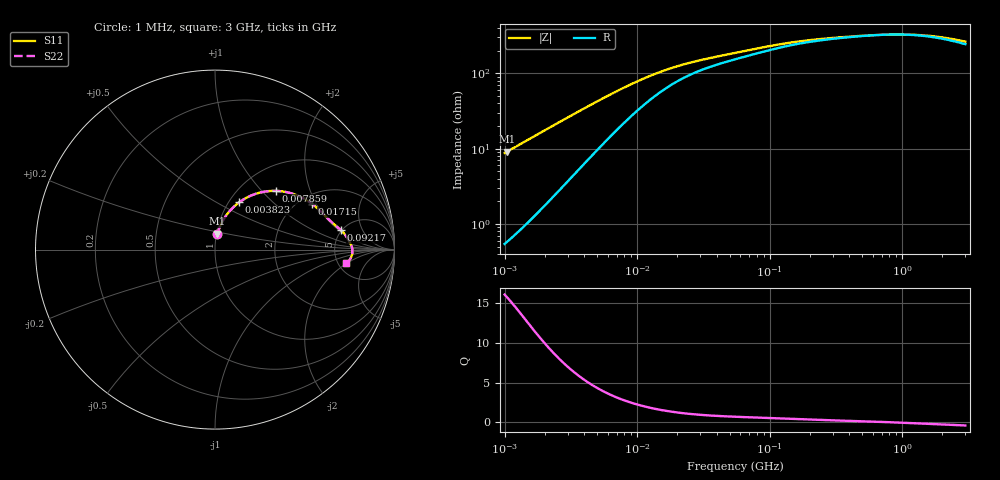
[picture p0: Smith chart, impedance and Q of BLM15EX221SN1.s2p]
! BLM15EX221SN1
# Hz S RI R 50
!Freq.(Hz) S11(Real) S11(Imag) S21(Real) S21(Imag) S12(Real) S12(Imag) S22(Real) S22(Imag)
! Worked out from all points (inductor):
!   401 points, 1 MHz to 3 GHz, reference 50 ohm
!   read as one part in series: L = 1.39 uH near 1.041 MHz
!   highest Q = 15.8 at 1.041 MHz (marker M1), where L = 1.39 uH
!   self-resonance near 817 MHz
!   S11 on the Smith chart (normalised r, x): 1 MHz: 1.01, +0.17; 3.823 MHz: 1.12, +0.65; 7.859 MHz: 1.43, +1.20; 17.15 MHz: 2.32, +1.84; 92.17 MHz: 4.92, +2.15; 3 GHz: 5.87, -1.96
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1000000  0.0128 0.0856  0.9872 -0.0856  0.9872 -0.0856  0.0128 0.0856
1040844  0.0138 0.089  0.9862 -0.089  0.9862 -0.089  0.0138 0.089
1553251  0.0283 0.1298  0.9717 -0.1298  0.9717 -0.1298  0.0283 0.1298
2182827  0.0524 0.1752  0.9476 -0.1752  0.9476 -0.1752  0.0524 0.1752
2947212  0.0885 0.2222  0.9115 -0.2222  0.9115 -0.2222  0.0885 0.2222
3823119  0.1354 0.2639  0.8646 -0.2639  0.8646 -0.2639  0.1354 0.2639
5705239  0.2384 0.3144  0.7616 -0.3144  0.7616 -0.3144  0.2384 0.3144
7858845  0.3382 0.3272  0.6618 -0.3272  0.6618 -0.3272  0.3382 0.3272
1.040059e7  0.4234 0.314  0.5766 -0.314  0.5766 -0.314  0.4234 0.314
1.461624e7  0.5085 0.2765  0.4915 -0.2765  0.4915 -0.2765  0.5085 0.2765
1.71545e7  0.5397 0.2554  0.4603 -0.2554  0.4603 -0.2554  0.5397 0.2554
2.718395e7  0.6031 0.1986  0.3969 -0.1986  0.3969 -0.1986  0.6031 0.1986
5.477226e7  0.6639 0.141  0.3361 -0.141  0.3361 -0.141  0.6639 0.141
9.216659e7  0.7014 0.1086  0.2986 -0.1086  0.2986 -0.1086  0.7014 0.1086
1.403209e8  0.7246 0.0829  0.2754 -0.0829  0.2754 -0.0829  0.7246 0.0829
2.094008e8  0.7395 0.0609  0.2605 -0.0609  0.2605 -0.0609  0.7395 0.0609
4.304467e8  0.7566 0.0291  0.2434 -0.0291  0.2434 -0.0291  0.7566 0.0291
8.005644e8  0.7653 0.00103  0.2347 -0.00103  0.2347 -0.00103  0.7653 0.00103
1.125055e9  0.7655 -0.0172  0.2345 0.0172  0.2345 0.0172  0.7655 -0.0172
1.54974e9  0.7611 -0.0362  0.2389 0.0362  0.2389 0.0362  0.7611 -0.0362
2.092429e9  0.7514 -0.0552  0.2486 0.0552  0.2486 0.0552  0.7514 -0.0552
3e9  0.7308 -0.077  0.2692 0.077  0.2692 0.077  0.7308 -0.077
